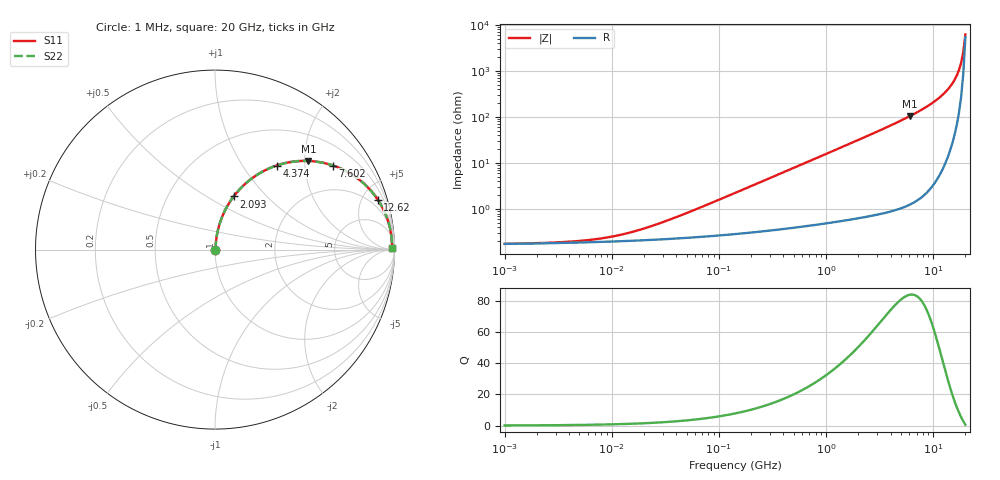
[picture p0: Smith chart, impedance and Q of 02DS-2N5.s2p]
# MHz S MA R 50
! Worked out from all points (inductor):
!   216 points, 1 MHz to 20 GHz, reference 50 ohm
!   read as one part in series: L = 2.5 nH near 45.75 MHz
!   highest Q = 83.6 at 6.038 GHz (marker M1), where L = 2.74 nH
!   S11 on the Smith chart (normalised r, x): 1 MHz: 1.00, +0.00; 2.093 GHz: 1.01, +0.66; 4.374 GHz: 1.02, +1.44; 7.602 GHz: 1.03, +2.78; 12.62 GHz: 1.17, +6.48; 20 GHz: open
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1  0.001756 5.1  0.9983 -0.0  0.9983 -0.0  0.001756 5.1
5.25016  0.002052 23.6  0.9981 -0.0  0.9981 -0.0  0.002052 23.6
12.0298  0.002749 43.2  0.998 -0.1  0.998 -0.1  0.002749 43.2
27.5642  0.004839 63.0  0.9978 -0.2  0.9978 -0.2  0.004839 63.0
144.716  0.02284 81.5  0.9969 -1.3  0.9969 -1.3  0.02284 81.5
363.591  0.05695 83.1  0.9948 -3.3  0.9948 -3.3  0.05695 83.1
759.783  0.1182 81.1  0.9886 -6.8  0.9886 -6.8  0.1182 81.1
1382.78  0.2122 76.3  0.9719 -12.2  0.9719 -12.2  0.2122 76.3
2093.13  0.3136 70.6  0.9435 -18.3  0.9435 -18.3  0.3136 70.6
2889.54  0.4179 64.4  0.9018 -24.7  0.9018 -24.7  0.4179 64.4
3988.98  0.5428 56.4  0.8325 -32.9  0.8325 -32.9  0.5428 56.4
4373.93  0.5811 53.7  0.8063 -35.5  0.8063 -35.5  0.5811 53.7
6038.17  0.717 43.5  0.6886 -45.8  0.6886 -45.8  0.717 43.5
7602.03  0.8071 35.5  0.5805 -53.8  0.5805 -53.8  0.8071 35.5
10022.1  0.8961 25.4  0.4297 -63.6  0.4297 -63.6  0.8961 25.4
12617.8  0.9486 17.0  0.2928 -71.5  0.2928 -71.5  0.9486 17.0
15170.5  0.9745 10.3  0.1796 -76.7  0.1796 -76.7  0.9745 10.3
16634.5  0.9821 7.0  0.1227 -78.1  0.1227 -78.1  0.9821 7.0
17418.7  0.9845 5.4  0.09425 -77.8  0.09425 -77.8  0.9845 5.4
18239.8  0.9859 3.7  0.06607 -75.9  0.06607 -75.9  0.9859 3.7
19099.6  0.9865 2.1  0.03858 -68.5  0.03858 -68.5  0.9865 2.1
20000  0.9862 0.4  0.01588 -29.1  0.01588 -29.1  0.9862 0.4
